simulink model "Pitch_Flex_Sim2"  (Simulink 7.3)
settings: Solver=ode45  StartTime=0.0  StopTime=120  FixedStep=0.01  RelTol=1e-3
InitFcn:
  | r2d= 180/pi; d2r=1/r2d; Ts=0.04;
  | [Apf,Bpf,Cpf,Dpf]= pitch_vehi_flex;              % Shuttle Ascent, Max_Q, T=55 sec, Flex Pitch Vehicle with Slosh and TWD
  | [Aac,Bac,Cac,Dac]= ssme_actuator;                % Shuttle Main Engine Actuator
  | [Asb,Bsb,Csb,Dsb]= srb_actuator;                 % Solid Rocket Booster Actuator
  | [Afc,Bfc,Cfc,Dfc]= pitch_fcs;                    % Pitch Axis Discrete FCS
  | [Apl,Bpl,Cpl,Dpl]= pitch_plant_s;                % Pitch Plant (Flex Vehicle, Actuators, TVC, TWD)
  | [Apz,Bpz,Cpz,Dpz]= pitch_plant_z;                % Pitch Plant Discrete
  | [Aol,Bol,Col,Dol]= open_loop;                    % Open-Loop Pitch (Plant Model + Controller)
  | [Acl,Bcl,Ccl,Dcl]= closed_loop;                  % Closed Loop (Plant Model + Controller)
StopFcn:
  | pl2
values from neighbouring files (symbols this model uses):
  Apl = [    [plant.m]    (also in plant_z.m)
  Bpl = [    [plant.m]    (also in plant_z.m)
  Cpl = [    [plant.m]    (also in plant_z.m)
  Dpl = [    [plant.m]    (also in plant_z.m)
undefined symbols (not defined in the file or in its folder): Afc, Bfc, Cfc, Dfc

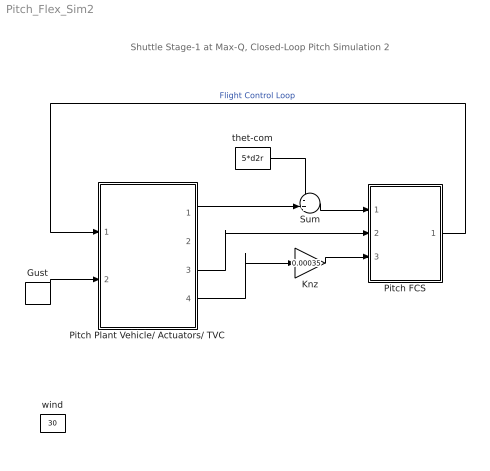
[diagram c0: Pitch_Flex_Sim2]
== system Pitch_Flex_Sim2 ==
  note: Shuttle Stage-1 at Max-Q, Closed-Loop Pitch Simulation 2
  Gust : DiscretePulseGenerator  PulseType=Time based  Amplitude=30  Period=200  PulseWidth=5  PhaseDelay=0.5  SampleTime=1
  Knz : Gain  Gain=0.00035  ParameterDataType=sfix(16)  ParameterScaling=2^0  OutDataType=sfix(16)  OutScaling=2^0
  Pitch FCS : Subsystem
  Pitch Plant Vehicle/ Actuators/ TVC : Subsystem
  Sum : Sum  Inputs=-+|  OutDataType=sfix(16)  OutScaling=2^0
  thet-com : Constant  Value=5*d2r  OutDataType=sfix(16)  OutScaling=2^0
  wind : Constant  Value=30  OutDataType=sfix(16)  OutScaling=2^0
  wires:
  Knz/1 -> Pitch FCS/3(Nz)
  Sum/1 -> Pitch FCS/1(theta)
  thet-com/1 -> Sum/1
  Pitch Plant Vehicle/ Actuators/ TVC/1(theta) -> Sum/2
  Pitch Plant Vehicle/ Actuators/ TVC/3(q-flx) -> Pitch FCS/2(q)
  Pitch Plant Vehicle/ Actuators/ TVC/4(Nz) -> Knz/1
  Pitch FCS/1(DQ_TVC) -> Pitch Plant Vehicle/ Actuators/ TVC/1(delt-c)  "Flight Control Loop"
  Gust/1 -> Pitch Plant Vehicle/ Actuators/ TVC/2(gust)

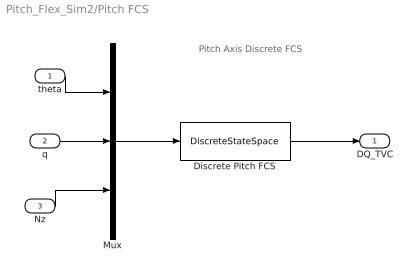
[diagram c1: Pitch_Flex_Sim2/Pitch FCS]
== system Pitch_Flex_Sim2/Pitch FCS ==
  note: Pitch Axis Discrete FCS
  theta : Inport  OutDataType=sfix(16)  OutScaling=2^0
  q : Inport  Port=2  OutDataType=sfix(16)  OutScaling=2^0
  Nz : Inport  Port=3  OutDataType=sfix(16)  OutScaling=2^0
  Discrete Pitch FCS : DiscreteStateSpace  A=Afc  B=Bfc  C=Cfc  D=Dfc  SampleTime=Ts
  Mux : Mux  Inputs=3
  DQ_TVC : Outport  OutDataType=sfix(16)  OutScaling=2^0
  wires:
  Discrete Pitch FCS/1 -> DQ_TVC/1
  theta/1 -> Mux/1
  q/1 -> Mux/2
  Nz/1 -> Mux/3
  Mux/1 -> Discrete Pitch FCS/1

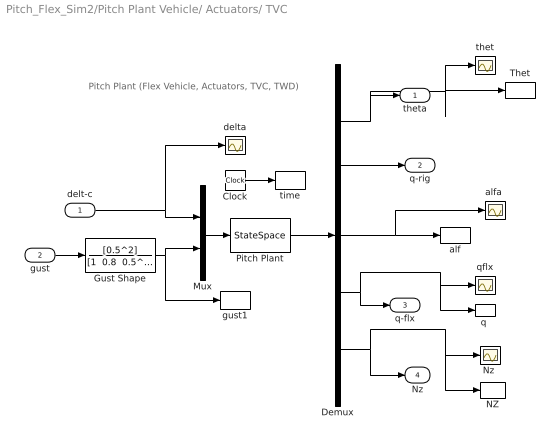
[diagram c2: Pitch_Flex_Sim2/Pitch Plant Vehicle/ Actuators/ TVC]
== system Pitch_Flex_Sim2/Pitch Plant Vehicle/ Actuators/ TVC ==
  note: Pitch Plant (Flex Vehicle, Actuators, TVC, TWD)
  delt-c : Inport  OutDataType=sfix(16)  OutScaling=2^0
  gust : Inport  Port=2  OutDataType=sfix(16)  OutScaling=2^0
  Clock : Clock
  Demux : Demux  Outputs=5
  Gust Shape : TransferFcn  Numerator=[0.5^2]  Denominator="[1  0.8  0.5^2]"
  Mux : Mux  Inputs=2
  NZ : ToWorkspace  VariableName=Nz  SampleTime=-1  SaveFormat=Array
  "Nz " : Scope
  Pitch Plant : StateSpace  A=Apl  B=Bpl  C=Cpl  D=Dpl
  Thet : ToWorkspace  VariableName=theta  SampleTime=-1  SaveFormat=Array
  alf : ToWorkspace  VariableName=alpha  SampleTime=-1  SaveFormat=Array
  "alfa " : Scope
  delta : Scope
  gust1 : ToWorkspace  VariableName=Gust  SampleTime=-1  SaveFormat=Array
  "q " : ToWorkspace  VariableName=q  SampleTime=-1  SaveFormat=Array
  qflx : Scope
  thet : Scope
  time : ToWorkspace  VariableName=time  SampleTime=-1  SaveFormat=Array
  theta : Outport  OutDataType=sfix(16)  OutScaling=2^0
  q-rig : Outport  Port=2  OutDataType=sfix(16)  OutScaling=2^0
  q-flx : Outport  Port=3  OutDataType=sfix(16)  OutScaling=2^0
  Nz : Outport  Port=4  OutDataType=sfix(16)  OutScaling=2^0
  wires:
  Pitch Plant/1 -> Demux/1
  Mux/1 -> Pitch Plant/1
  delt-c/1 -> Mux/1, delta/1
  gust/1 -> Gust Shape/1
  Demux/1 -> theta/1, thet/1, Thet/1
  Demux/3 -> alf/1, "alfa "/1
  Demux/4 -> q-flx/1, qflx/1, "q "/1
  Demux/2 -> q-rig/1
  Demux/5 -> Nz/1, "Nz "/1, NZ/1
  Clock/1 -> time/1
  Gust Shape/1 -> Mux/2, gust1/1
